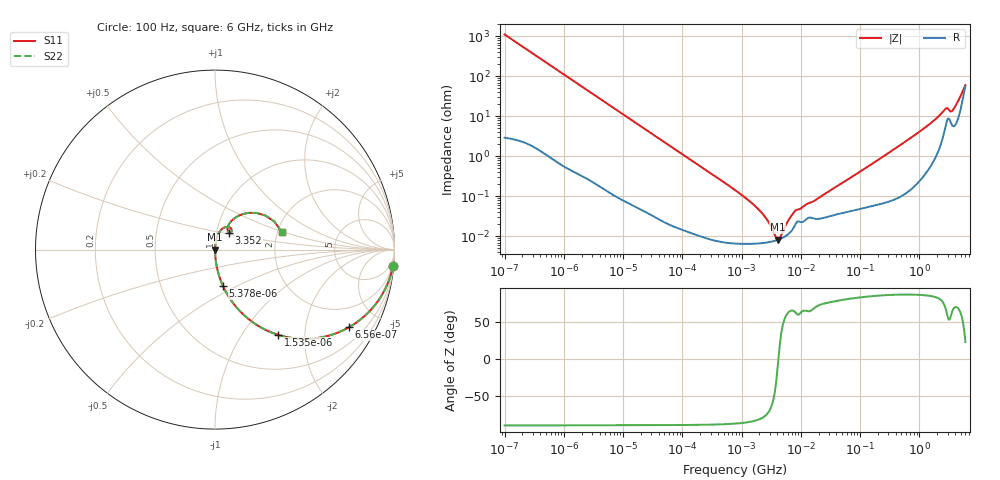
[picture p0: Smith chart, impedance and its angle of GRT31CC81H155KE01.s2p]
!Murata Part Number: GRT31CC81H155KE01
!These Parameters are Measured in Series Mode Connection
!Data Generated on Jun 19, 2026
!  o--ll--o
!Port1  Port2
!  o------o
!Operation Temp=25[degC], DC Bias Voltage=0[V]
!Freq. Start=100[Hz] Stop=6[GHz] 401[Steps]
# Hz S RI R 50
!Freq.(Hz) S11(Real) S11(Imag) S21(Real) S21(Imag) S12(Real) S12(Imag) S22(Real) S22(Imag)
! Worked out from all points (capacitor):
!   401 points, 100 Hz to 6 GHz, reference 50 ohm
!   read as one part in series: C = 1.42 uF near 109 Hz
!   lowest |Z| = 8.37 mohm at 4.06 MHz (marker M1)
!   series resonance near 4.183 MHz, so ESL is about 1 nH
!   S11 on the Smith chart (normalised r, x): 100 Hz: 1, -22; 656 Hz: 1.02, -3.43; 1.535 kHz: 1.01, -1.47; 5.378 kHz: 1.00, -0.42; 3.352 GHz: 1.15, +0.22; 6 GHz: 2.12, +0.48
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100  0.9918 -0.0887  0.00816 0.0887  0.00816 0.0887  0.9918 -0.0887
306  0.9296 -0.2535  0.0704 0.2535  0.0704 0.2535  0.9296 -0.2535
656  0.7453 -0.4332  0.2547 0.4332  0.2547 0.4332  0.7453 -0.4332
1535  0.3512 -0.4746  0.6488 0.4746  0.6488 0.4746  0.3512 -0.4746
2008  0.2413 -0.425  0.7587 0.425  0.7587 0.425  0.2413 -0.425
5378  0.0437 -0.2012  0.9563 0.2012  0.9563 0.2012  0.0437 -0.2012
40335  0.00107 -0.0283  0.9989 0.0283  0.9989 0.0283  0.00107 -0.0283
774597  6.85e-05 -0.00144  0.9999 0.00144  0.9999 0.00144  6.85e-05 -0.00144
2074311  6.76e-05 -0.000421  0.9999 0.000421  0.9999 0.000421  6.76e-05 -0.000421
4060267  8.21e-05 -1.65e-05  0.9999 1.65e-05  0.9999 1.65e-05  8.21e-05 -1.65e-05
4643984  8.88e-05 5.86e-05  0.9999 -5.86e-05  0.9999 -5.86e-05  8.88e-05 5.86e-05
6353432  0.000119 0.000244  0.9999 -0.000244  0.9999 -0.000244  0.000119 0.000244
7947587  0.000189 0.000384  0.9998 -0.000384  0.9998 -0.000384  0.000189 0.000384
1.555665e7  0.00029 0.000669  0.9997 -0.000669  0.9997 -0.000669  0.00029 0.000669
3.124326e8  0.000907 0.0126  0.9991 -0.0126  0.9991 -0.0126  0.000907 0.0126
1.309207e9  0.00689 0.0546  0.9931 -0.0546  0.9931 -0.0546  0.00689 0.0546
2.679998e9  0.0603 0.1261  0.9397 -0.1261  0.9397 -0.1261  0.0603 0.1261
3.352442e9  0.0788 0.0946  0.9212 -0.0946  0.9212 -0.0946  0.0788 0.0946
3.666503e9  0.0688 0.115  0.9312 -0.115  0.9312 -0.115  0.0688 0.115
4.385646e9  0.1055 0.1725  0.8945 -0.1725  0.8945 -0.1725  0.1055 0.1725
5.245841e9  0.2307 0.2042  0.7693 -0.2042  0.7693 -0.2042  0.2307 0.2042
6e9  0.3732 0.0958  0.6268 -0.0958  0.6268 -0.0958  0.3732 0.0958
